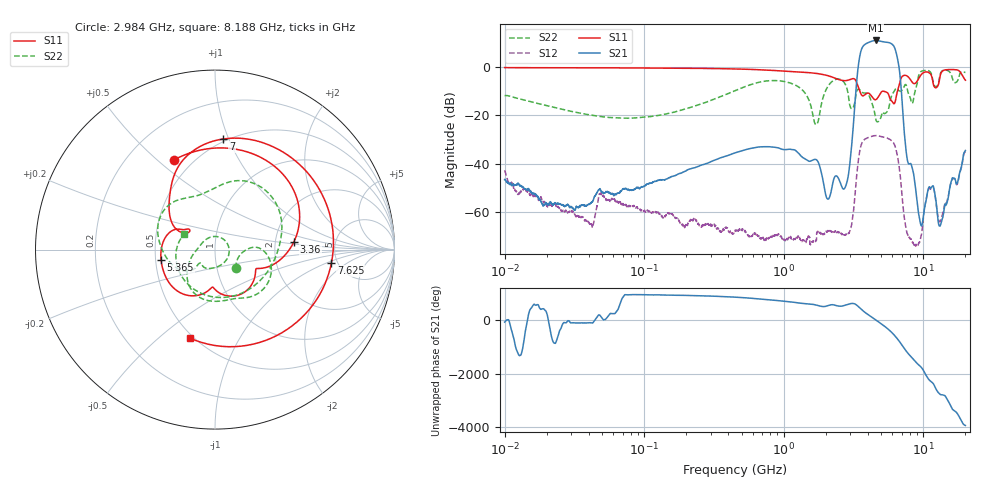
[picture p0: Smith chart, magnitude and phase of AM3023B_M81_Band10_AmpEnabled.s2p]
!Agilent Technologies,E8364B,MY43040894,A.07.50.67
!Agilent E8364B: A.07.50.67
!Date: Tuesday, October 27, 2020 10:45:22
!Correction: S11(Full 2 Port(1,2))
!S21(Full 2 Port(1,2))
!S12(Full 2 Port(1,2))
!S22(Full 2 Port(1,2))
!S2P File: Measurements: S11, S21, S12, S22:Log Frequency Sweep
# Hz S  dB  R 50
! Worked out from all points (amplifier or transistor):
!   3201 points, 10 MHz to 20 GHz, reference 50 ohm
!   highest |S21| = 10.9 dB at 4.554 GHz (marker M1)
!   |S21| within 3 dB of that: 3.644 GHz to 6.221 GHz (2.577 GHz wide, 52.2 % of centre)
!   unconditionally stable (mu >= 1): start of sweep to end of sweep
!   at 35.47 MHz: K = 35544.81, MAG = -46.1 dB, |S12| = -61.9 dB
!   at 447.2 MHz: K = 12131.88, MAG = -27.5 dB, |S12| = -68.3 dB
!   at 20 GHz: K = 436.46, MAG = -29.2 dB, |S12| = -34.9 dB
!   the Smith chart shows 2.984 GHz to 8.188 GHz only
!   S11 on the Smith chart (normalised r, x): 2.984 GHz: 0.40, +0.57; 3.36 GHz: 2.55, +0.28; 5.365 GHz: 0.53, -0.07; 7 GHz: 0.48, +0.96; 7.625 GHz: 4.45, -1.14; 8.188 GHz: 0.48, -0.64
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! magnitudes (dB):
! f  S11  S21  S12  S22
! 10 MHz  -0.3  -46.6  -42.7  -11.9
! 35.55 MHz  -0.4  -57.1  -62.0  -19.2
! 49.22 MHz  -0.4  -51.6  -52.8  -20.5
! 126.1 MHz  -0.5  -46.8  -60.2  -20.0
! 447.2 MHz  -0.8  -35.5  -68.3  -9.8
! 1.069 GHz  -1.8  -34.1  -71.3  -6.4
! 1.59 GHz  -2.5  -38.7  -72.5  -17.9
! 1.728 GHz  -2.7  -38.5  -68.6  -23.7
! 2.074 GHz  -3.6  -54.7  -67.7  -8.0
! 2.984 GHz  -5.2  -39.2  -67.6  -16.2
! 3.36 GHz  -7.1  -3.5  -42.6  -9.6
! 4.554 GHz  -13.5  10.9  -28.4  -21.6
! 5.365 GHz  -10.3  10.3  -29.2  -19.1
! 5.639 GHz  -11.4  10.1  -29.7  -17.2
! 6.426 GHz  -11.6  5.2  -35.1  -8.9
! 7 GHz  -4.2  -12.0  -52.0  -9.7
! 7.625 GHz  -3.7  -37.5  -68.5  -8.6
! 8.188 GHz  -5.8  -40.3  -71.3  -14.3
! 9.577 GHz  -3.4  -65.3  -70.5  -2.0
! 11.2 GHz  -2.8  -50.0  -50.4  -2.1
! 13.2 GHz  -3.6  -65.7  -63.8  -3.0
! 20 GHz  -5.5  -34.5  -34.9  -2.3
